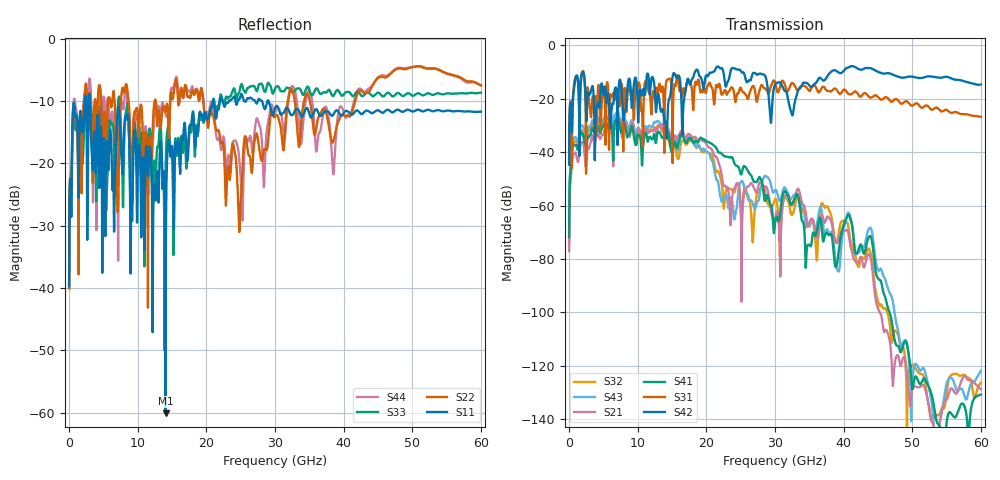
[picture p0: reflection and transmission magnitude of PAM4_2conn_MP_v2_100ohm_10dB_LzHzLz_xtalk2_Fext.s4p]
! Info: Touchstone file created by Circ.  Input file=FAB50GbE_2conn_Midplane_Examax_Topo2_v2_100ohm_10dB_LzHzLz.circ
# Hz S RI R 50
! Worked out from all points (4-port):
!   6000 points, 10 MHz to 60 GHz, reference 50 ohm
!   strongest paths, dB at 10 MHz, 15.01 GHz, 30.01 GHz, 45.01 GHz, 60 GHz:
!     S42: -44.7, -13.0, -14.7, -9.9, -14.7
!     S31: -44.0, -22.3, -13.9, -19.4, -26.8
!     S41: -71.8, -37.8, -66.3, -87.2, -130.8
!     S21: -77.1, -35.3, -66.0, -98.5, -128.8
!     S43: -71.9, -35.0, -54.3, -84.1, -121.9
!     S32: -73.7, -38.4, -57.7, -95.7, -126.4
!   lowest |S11| = -60.1 dB at 14.06 GHz (marker M1), VSWR 1.00, Z = 49.9 - j0.0622 ohm
!   |S11| at or under -10 dB: start of sweep to 2.295 GHz; 3.042 GHz to 21.01 GHz (17.97 GHz wide, 149 % of centre); 29.06 GHz to end of sweep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
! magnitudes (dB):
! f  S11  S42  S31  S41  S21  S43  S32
! 10 MHz  -39.7  -44.7  -44.0  -71.8  -77.1  -71.9  -73.7
! 1.86 GHz  -14.1  -10.4  -10.8  -32.7  -36.2  -30.0  -31.7
! 14.06 GHz  -60.1  -28.6  -15.6  -31.0  -30.6  -29.2  -31.3
! 15.34 GHz  -24.3  -10.5  -14.7  -36.7  -34.3  -35.0  -37.9
! 24.85 GHz  -9.7  -9.1  -16.3  -46.7  -54.5  -52.1  -55.3
! 39.05 GHz  -11.5  -9.8  -16.9  -81.7  -74.0  -84.0  -73.5
! 60 GHz  -11.7  -14.7  -26.8  -130.8  -128.8  -121.9  -126.4
